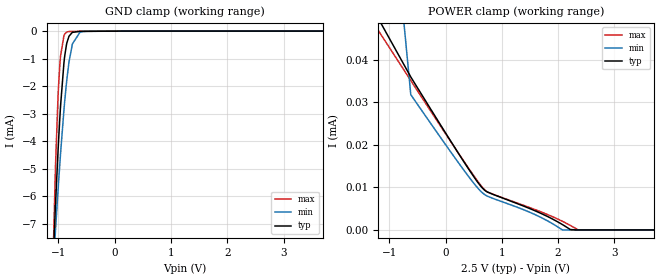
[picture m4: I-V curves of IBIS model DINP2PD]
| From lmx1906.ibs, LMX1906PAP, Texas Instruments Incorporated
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|   Model DINP2PD
[Model]   DINP2PD
Model_type   Input
Vinl = 0.4
Vinh = 1.4
|   typ   min   max
C_comp   0.0195pF   0.0186pF   0.0315pF
[Voltage Range]   2.5   2.4   2.6
[Temperature Range]   27   105   -40
[Power Clamp Reference]   2.5   2.4   2.6
[GND Clamp Reference]   0   0   0
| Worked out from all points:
|   GND clamp passes 1 mA (typ) near -0.89 V on its own axis
|   POWER clamp passes 1 mA (typ) near -1.77 V on its own axis
[GND Clamp]
|   Voltage   I(typ)   I(min)   I(max)
-2.5V     -99.58mA   -67.34mA   -181.2mA
-1.113V   -9.254mA   -9.296mA   -9.568mA
-1.052V   -6.307mA   -7.24mA    -4.898mA
-1.008V   -4.357mA   -5.791mA   -2.386mA
-977.5mV  -3.224mA   -4.882mA   -1.284mA
-962.5mV  -2.717mA   -4.447mA   -899.9uA
-902.5mV  -1.154mA   -2.866mA   -170.3uA
-850mV    -423.7uA   -1.743mA   -33.67uA
-812.5mV  -185.3uA   -1.122mA   -15.04uA
-752.5mV  -45.96uA   -468.4uA   -10.53uA
-572.5mV  -9.365uA   -19.6uA    -8.135uA
5V        0A         0A         0A
[POWER Clamp]
|   Voltage   I(typ)   I(min)   I(max)
-2.5V     12.94mA    14.08mA    11.82mA
-1.337V   53.17uA    131.6uA    49.86uA
-617.5mV  36.01uA    31.84uA    35.17uA
432.5mV   13.89uA    12.18uA    14.08uA
627.5mV   10.28uA    9.088uA    10.48uA
747.5mV   8.917uA    7.928uA    8.918uA
1.573V    4.616uA    3.726uA    4.887uA
2.075V    1.287uA    29.17nA    2.051uA
2.217V    104.2nA    0A         1.071uA
2.353V    0A         0A         48.87nA
2.428V    0A         0A         0A
5V        0A         0A         0A
